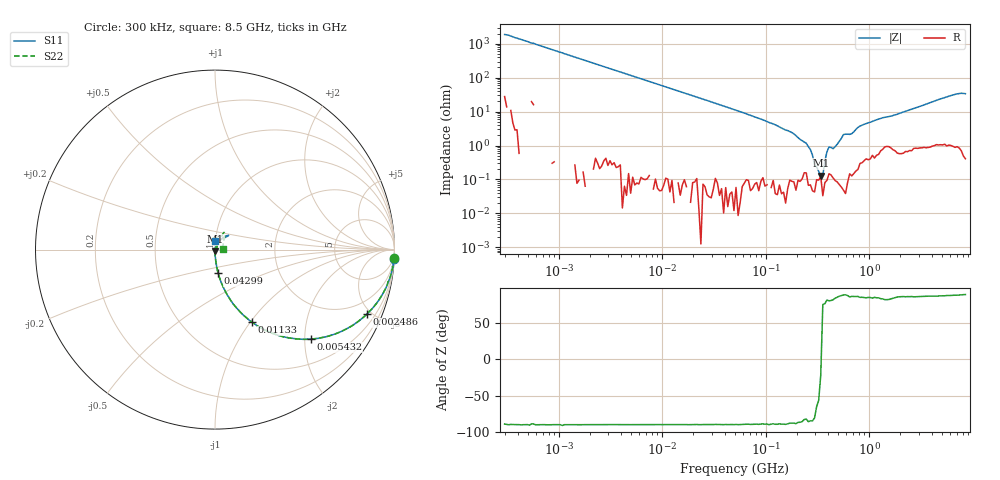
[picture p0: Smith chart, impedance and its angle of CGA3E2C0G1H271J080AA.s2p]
! S-parameter Generated by TDK Corporation
! Copyright(C) 2015 TDK Corporation.
! All Rights Reserved.
! TDK P/N: CGA3E2C0G1H271J080AA (Multilayer Ceramic Chip Capacitors)
! Property: C=270pF
! Size(LxWxT): 1.6x0.8x0.8mm, 0.063x0.031x0.031inches
! Model Type: s2p (Touchstone File Format Version 1.0)
! Frequency: DC=Yes Start=0.3MHz Stop=8500MHz 225points Log-sweep
! Note:
! Model Generated on Jun. 23, 2015
! Hash(MD5):
! Port Assignments:
!  1 ---| |--- 2
! Applicable Conditions:
!  Temperature = 25 degC
!  DC Bias Voltage = 0 V
!  Small Signal Operation
! Terms and conditions regarding TDK Simulation Models
! (1)This simulation model is being provided solely for informational purposes. Please refer to the specifications of the products in terms of detailed characteristics of such products.
! (2)In no event shall TDK Corporation of any of its subsidiaries be liable for any loss or damage arising, directly or indirectly,
!  From any information contained in this simulation model, including, but not limited to loss or damages arising from any inaccuracies, omissions or errors in connection with such information.
! (3)Any and all copyrights on this simulation model are owned by TDK Corporation.
!  Duplication or redistribution of this simulation model without prior written permission from TDK Corporation is prohibited.
! (4)This simulation model is subject to any modification or change without any prior notice.
! (5)Neither TDK Corporation nor any of its subsidiaries shall make any warranty, express or implied,
!  Including but not limited to the correctness, implied warranties of merchantability and fitness for a particular purpose with respect to this simulation models.
! (6)The use of this simulation model shall be deemed to have consented to the terms and conditions hereof.
# MHz S MA R 50
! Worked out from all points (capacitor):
!   224 points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, 300 kHz to 8.5 GHz, reference 50 ohm
!   read as one part in series: C = 274 pF near 314.1 kHz
!   lowest |Z| = 130 mohm at 340.3 MHz (marker M1)
!   series resonance near 344.7 MHz, so ESL is about 780 pH
!   S11 on the Smith chart (normalised r, x): 300 kHz: 2, -39; 2.486 MHz: 1.01, -4.68; 5.432 MHz: 1.00, -2.14; 11.33 MHz: 1.00, -1.02; 42.99 MHz: 1.00, -0.27; 8.5 GHz: 1.00, +0.10
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0.3  0.9977 -2.9  0.05297 86.3  0.05235 86.1  0.9976 -2.7
1.72111  0.9579 -16.5  0.2845 73.5  0.284 73.4  0.9586 -16.5
2.486179  0.9187 -23.1  0.3937 66.8  0.3938 66.8  0.919 -23.1
5.431819  0.7293 -43.1  0.6832 46.9  0.6831 46.9  0.73 -43.1
9.430415  0.5239 -58.4  0.8516 31.5  0.8515 31.6  0.524 -58.4
11.33425  0.4555 -62.9  0.8896 27.0  0.8888 27.0  0.4559 -62.9
42.99233  0.1331 -82.4  0.991 7.5  0.9908 7.5  0.133 -82.5
51.67171  0.1106 -83.4  0.9931 6.2  0.9933 6.1  0.1105 -83.6
283.1228  0.0138 -87.5  0.9997 -0.2  0.9991 -0.2  0.01345 -89.5
340.2802  0.01032 -83.1  0.9986 -0.5  0.9973 -0.4  0.008502 -93.4
408.9767  0.004536 -81.0  0.9974 -1.3  0.9978 -1.3  0.004605 -87.1
469.456  0.003338 -62.2  0.9994 -1.2  0.9983 -1.2  0.001657 -96.7
514.6664  0.000952 -16.1  0.9991 -1.6  0.9986 -1.5  0.0006967 -130.1
564.2308  0.001246 27.2  0.9992 -2.3  0.9986 -2.3  0.002931 113.4
618.5683  0.003747 64.4  0.9991 -2.3  0.9987 -2.3  0.002655 94.1
815.0429  0.009401 79.2  0.9965 -3.7  0.9967 -3.8  0.009509 61.7
1177.346  0.0159 74.9  0.9943 -5.6  0.9944 -5.7  0.01728 61.2
1551.304  0.01633 57.9  0.9899 -7.3  0.9897 -7.2  0.01789 49.6
2240.89  0.02176 69.0  0.9926 -10.5  0.9913 -10.5  0.0212 60.7
6450.987  0.1081 46.9  0.9823 -30.6  0.9832 -30.6  0.1063 62.8
7753.325  0.09353 48.6  0.9831 -36.5  0.9857 -36.6  0.08978 53.1
8500  0.04983 88.1  0.9854 -39.8  0.9877 -39.7  0.0422 6.7
